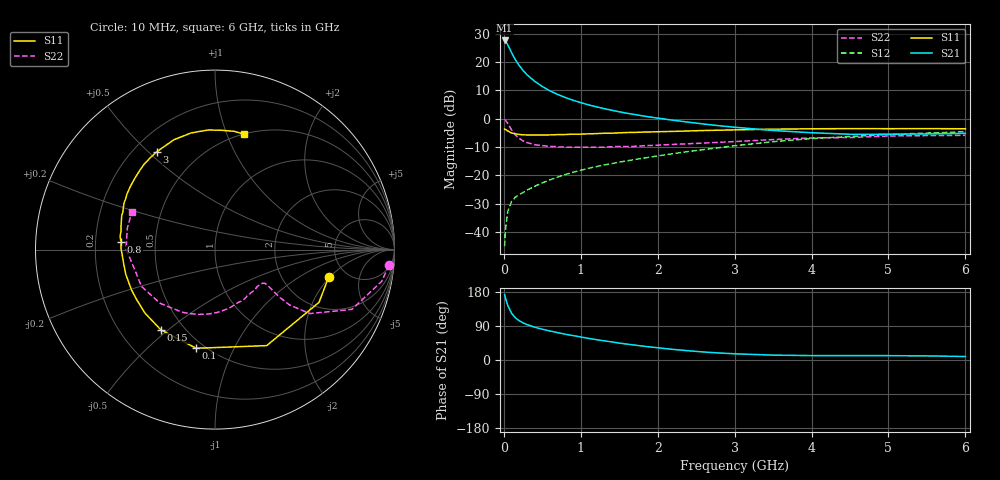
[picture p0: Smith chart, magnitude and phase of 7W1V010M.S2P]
! Infineon Technologies  Discrete & RF Semiconductors
! BFS17W
! Si NPN RF Bipolar Junction Transistor in SOT323
! VCE = 1 V  IC = 10 mA
! Common Emitter S-Parameters:  August  1999
# GHz  S  MA  R  50
!  f  S11  S21  S12  S22
! GHz  MAG  ANG  MAG  ANG  MAG  ANG  MAG  ANG
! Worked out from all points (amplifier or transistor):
!   36 points, 10 MHz to 6 GHz, reference 50 ohm
!   highest |S21| = 27.6 dB at 10 MHz (marker M1)
!   |S21| within 3 dB of that: start of sweep to 77.18 MHz
!   unconditionally stable (mu >= 1): 340.8 MHz to end of sweep
!   at 250 MHz: K = 0.86, MSG = 21.5 dB, |S12| = -26.1 dB
!   at 1.4 GHz: K = 1.31, MAG = 6.1 dB, |S12| = -15.9 dB
!   at 6 GHz: K = 1.12, MAG = -2.3 dB, |S12| = -4.6 dB
!   S11 on the Smith chart (normalised r, x): 10 MHz: 3.64, -1.94; 100 MHz: 0.45, -0.72; 150 MHz: 0.37, -0.47; 800 MHz: 0.31, +0.04; 3 GHz: 0.29, +0.53; 6 GHz: 0.50, +1.15
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0.01  0.6517 -13.6  24.11 172.6  0.0056 83.3  0.9738 -5.1
0.02  0.6498 -26.9  23.55 164.5  0.0104 80.1  0.9452 -10.8
0.05  0.6076 -61.7  20.36 144.6  0.0228 64.9  0.8321 -23.6
0.1  0.5597 -100.8  14.71 123.5  0.0345 52.3  0.6375 -34.0
0.15  0.5393 -124.0  11.02 111.3  0.041 48.4  0.5163 -36.6
0.2  0.5267 -137.8  8.687 103.6  0.0456 49.3  0.4484 -36.4
0.25  0.5179 -147.5  7.109 98.0  0.0498 49.4  0.4044 -35.6
0.3  0.5166 -154.4  6.008 93.6  0.0545 51.3  0.3796 -34.9
0.4  0.5158 -164.5  4.585 86.6  0.0639 54.1  0.3474 -34.1
0.5  0.5147 -171.2  3.701 81.2  0.0732 56.4  0.3342 -34.1
0.6  0.5172 -176.1  3.102 76.5  0.0833 58.0  0.3248 -35.2
0.7  0.5236 179.6  2.685 72.2  0.0931 59.6  0.3187 -37.1
0.8  0.5256 175.4  2.367 68.0  0.1033 60.1  0.3149 -39.5
1.1  0.5403 165.7  1.759 57.1  0.133 61.0  0.3138 -48.0
1.3  0.553 160.0  1.511 50.7  0.1521 60.8  0.314 -55.0
1.6  0.5701 152.6  1.249 41.9  0.18 60.7  0.3215 -65.8
2.2  0.5968 138.7  0.94 28.0  0.2412 59.4  0.3515 -88.5
3  0.6346 120.7  0.707 16.4  0.3326 54.4  0.3945 -117.9
3.5  0.6534 110.5  0.619 12.9  0.3924 49.4  0.4277 -135.6
4.5  0.6676 93.1  0.531 11.6  0.4838 37.2  0.4643 -168.4
5.5  0.6676 80.8  0.538 10.8  0.5571 26.1  0.5026 166.6
6  0.6634 75.9  0.552 9.2  0.5873 20.7  0.5087 155.6
